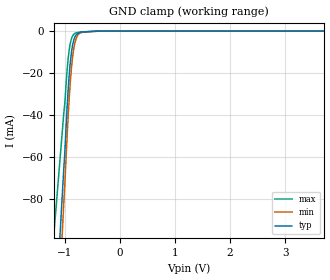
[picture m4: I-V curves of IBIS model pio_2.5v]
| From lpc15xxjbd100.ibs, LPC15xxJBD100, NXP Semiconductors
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[Model] pio_2.5v
Model_type Input
Vinl = 750.000mV
Vinh = 1.75000V
C_comp 598.000fF 598.000fF 598.000fF
| variable typ   min   max
[Voltage Range] 2.50000V 2.25000V 2.75000V
[POWER Clamp Reference] 2.50000V 2.25000V 2.75000V
[GND Clamp Reference] 0.00000V 0.00000V 0.00000V
[Temperature Range]   25   85   -40
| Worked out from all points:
|   GND clamp passes 1 mA (typ) near -0.75 V on its own axis
[GND Clamp]
-2.5V     -751.2mA   -845mA     -512.1mA
-1.02V    -65.72mA   -82.28mA   -39.39mA
-1V       -57.52mA   -72.74mA   -34.23mA
-960mV    -36.8mA    -50.53mA   -18.93mA
-940mV    -28mA      -40.54mA   -13.13mA
-900mV    -14.62mA   -23.94mA   -5.672mA
-860mV    -6.743mA   -12.52mA   -2.364mA
-840mV    -4.432mA   -8.664mA   -1.584mA
-800mV    -1.977mA   -3.9mA     -857.9uA
-700mV    -522.6uA   -703.6uA   -398.5uA
-320mV    0A         0A         0A
5V        0A         0A         0A
[Power Clamp]
-2.5V     0A         0A         0A
0V        0A         0A         0A
2.5V      0A         0A         0A
5V        0A         0A         0A
